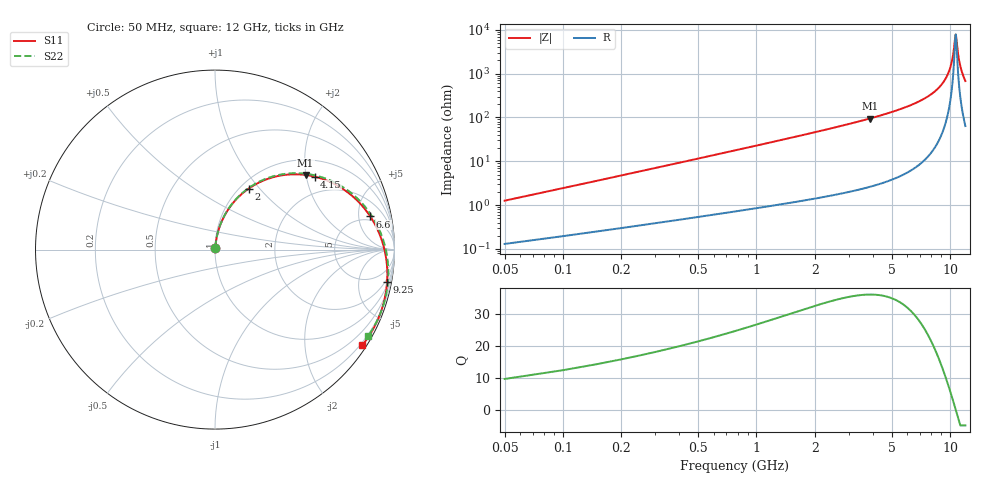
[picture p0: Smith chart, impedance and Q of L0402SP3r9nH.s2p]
!	AVX Thin Film Operation
!	Date:		5 January 2004
!	Description: 	Accu-L®  L0402 Series Thin Film RF Inductors
!	Part Number:	L04023R9BHLTR
!	50 MHz-20GHz Serial Measurements
#	mhz	S	db	R	50
!	S11	S11	S21	S21	S12	S12	S22	S22
!	dB	Phase	dB	Phase	dB	Phase	dB	Phase
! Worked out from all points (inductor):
!   240 points, 50 MHz to 12 GHz, reference 50 ohm
!   read as one part in series: L = 3.81 nH near 100 MHz
!   highest Q = 36.2 at 3.85 GHz (marker M1), where L = 3.92 nH
!   self-resonance near 10.65 GHz
!   S11 on the Smith chart (normalised r, x): 50 MHz: 1.00, +0.02; 2 GHz: 1.09, +0.87; 4.15 GHz: 1.45, +2.24; 6.6 GHz: 4.15, +7.05; 9.25 GHz: 1, -10; 12 GHz: 0.13, -3.37
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50  -38.58 82.9  -0.01 -0.8  -0.01 -0.8  -38.58 82.9
100  -32.90 83.5  -0.02 -1.5  -0.02 -1.5  -32.90 83.6
200  -27.15 83.2  -0.03 -2.9  -0.03 -2.9  -27.15 83.2
350  -22.49 81.7  -0.06 -5.0  -0.06 -5.0  -22.49 81.8
550  -18.71 79.4  -0.11 -7.7  -0.11 -7.7  -18.71 79.5
1150  -12.62 71.9  -0.33 -15.8  -0.33 -15.8  -12.62 72.1
2000  -8.23 61.2  -0.83 -26.7  -0.83 -26.7  -8.23 61.6
2050  -8.04 60.5  -0.86 -27.3  -0.86 -27.3  -8.04 61.0
3850  -3.69 39.5  -2.64 -48.4  -2.64 -48.4  -3.69 40.4
4050  -3.39 37.3  -2.89 -50.5  -2.89 -50.5  -3.39 38.2
4150  -3.25 36.2  -3.02 -51.6  -3.02 -51.6  -3.25 37.2
6050  -1.40 17.2  -6.07 -70.2  -6.07 -70.2  -1.40 18.6
6600  -1.07 12.1  -7.21 -75.1  -7.21 -75.1  -1.07 13.7
8050  -0.47 -0.7  -11.11 -86.9  -11.11 -86.9  -0.47 1.3
9250  -0.21 -10.7  -16.43 -94.7  -16.43 -94.7  -0.21 -8.4
10050  -0.13 -17.3  -23.38 -95.5  -23.38 -95.5  -0.13 -14.6
10350  -0.11 -19.7  -28.50 -89.3  -28.50 -89.3  -0.11 -17.0
10700  -0.11 -22.5  -38.29 -18.4  -38.29 -18.4  -0.11 -19.7
11000  -0.11 -25.0  -29.46 45.4  -29.46 45.4  -0.11 -22.0
11200  -0.12 -26.6  -25.47 51.8  -25.47 51.8  -0.12 -23.5
11550  -0.14 -29.4  -21.06 54.3  -21.06 54.3  -0.14 -26.2
12000  -0.19 -33.0  -17.46 53.5  -17.46 53.5  -0.18 -29.6
